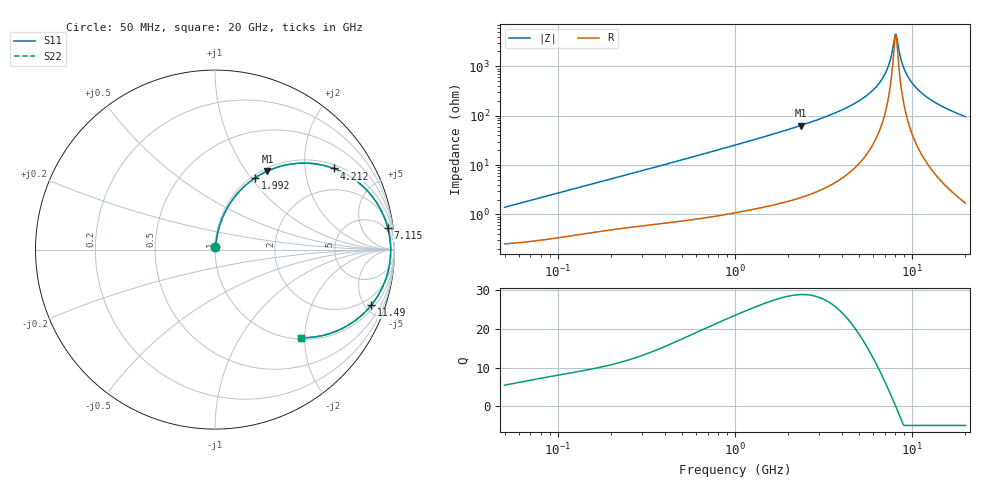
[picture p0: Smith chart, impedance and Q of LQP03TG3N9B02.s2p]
!Murata Part Number: LQP03TG3N9B02
!These Parameters are Measured in Series Mode Connection
!  o--[Z]--o
!Port1  Port2
!  o-------o
!Freq. Start=50[MHz] Stop=20[GHz], 401[Steps]
# Hz S RI R 50
!Freq.(Hz) S11(Real) S11(Imag) S21(Real) S21(Imag) S12(Real) S12(Imag) S22(Real) S22(Imag)
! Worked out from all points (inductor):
!   401 points, 50 MHz to 20 GHz, reference 50 ohm
!   read as one part in series: L = 4.35 nH near 51.52 MHz
!   highest Q = 28.9 at 2.349 GHz (marker M1), where L = 4.28 nH
!   self-resonance near 8.021 GHz
!   S11 on the Smith chart (normalised r, x): 50 MHz: 1.01, +0.03; 1.992 GHz: 1.04, +1.05; 4.212 GHz: 1.12, +2.83; 7.115 GHz: 4, +15; 11.49 GHz: 1.30, -5.49; 20 GHz: 1.03, -1.91
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5e7  0.0027 0.0136  0.9973 -0.0136  0.9973 -0.0136  0.0027 0.0136
1.364002e8  0.00525 0.0359  0.9947 -0.0359  0.9947 -0.0359  0.00525 0.0359
3.721004e8  0.0151 0.0929  0.9849 -0.0929  0.9849 -0.0929  0.0151 0.0929
1e9  0.069 0.2331  0.931 -0.2331  0.931 -0.2331  0.069 0.2331
1.99176e9  0.223 0.3991  0.777 -0.3991  0.777 -0.3991  0.223 0.3991
2.348516e9  0.2919 0.4376  0.7081 -0.4376  0.7081 -0.4376  0.2919 0.4376
2.728004e9  0.3689 0.4654  0.6311 -0.4654  0.6311 -0.4654  0.3689 0.4654
4.212059e9  0.6615 0.4522  0.3385 -0.4522  0.3385 -0.4522  0.6615 0.4522
5.041459e9  0.7911 0.3804  0.2089 -0.3804  0.2089 -0.3804  0.7911 0.3804
5.856089e9  0.8841 0.2853  0.1159 -0.2853  0.1159 -0.2853  0.8841 0.2853
6.503449e9  0.9338 0.2016  0.0662 -0.2016  0.0662 -0.2016  0.9338 0.2016
7.114996e9  0.9628 0.1213  0.0372 -0.1213  0.0372 -0.1213  0.9628 0.1213
7.442007e9  0.9721 0.0791  0.0279 -0.0791  0.0279 -0.0791  0.9721 0.0791
7.901521e9  0.9785 0.0217  0.0215 -0.0217  0.0215 -0.0217  0.9785 0.0217
8.141811e9  0.9791 -0.00731  0.0209 0.00731  0.0209 0.00731  0.9791 -0.00731
8.264682e9  0.9787 -0.0218  0.0213 0.0218  0.0213 0.0218  0.9787 -0.0218
8.774992e9  0.9731 -0.0795  0.0269 0.0795  0.0269 0.0795  0.9731 -0.0795
9.316812e9  0.9607 -0.1358  0.0393 0.1358  0.0393 0.1358  0.9607 -0.1358
1.019291e10  0.9303 -0.2158  0.0697 0.2158  0.0697 0.2158  0.9303 -0.2158
1.149051e10  0.8705 -0.3099  0.1295 0.3099  0.1295 0.3099  0.8705 -0.3099
1.460232e10  0.708 -0.44  0.292 0.44  0.292 0.44  0.708 -0.44
2e10  0.4778 -0.4908  0.5222 0.4908  0.5222 0.4908  0.4778 -0.4908
